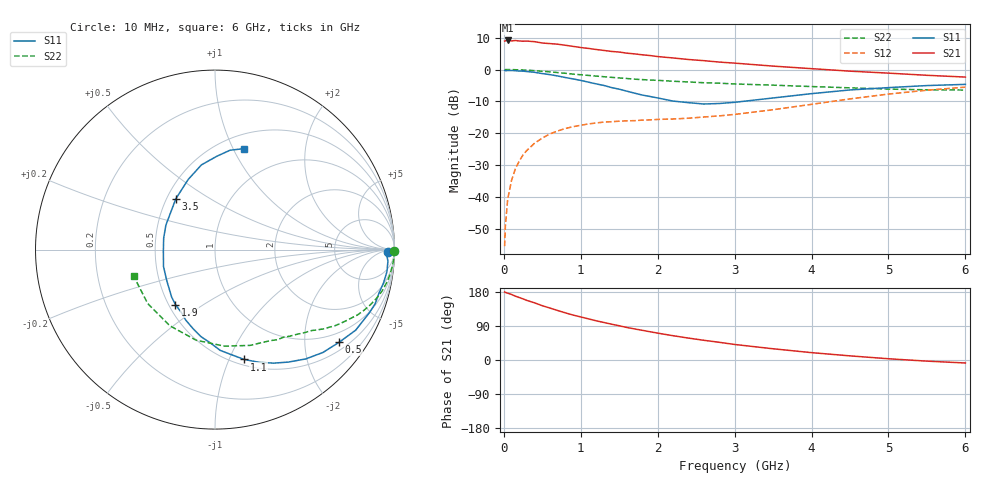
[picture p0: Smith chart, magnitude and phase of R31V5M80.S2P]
! SIEMENS Small Signal Semiconductors
! BFR181
! Si NPN RF Bipolar Junction Transistor in SOT23
! VCE = 1.5 V  IC = 0.8 mA
! Common Emitter S-Parameters:  May  1996
# GHz  S  MA  R  50
!  f  S11  S21  S12  S22
! GHz  MAG  ANG  MAG  ANG  MAG  ANG  MAG  ANG
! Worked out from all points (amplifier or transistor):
!   36 points, 10 MHz to 6 GHz, reference 50 ohm
!   highest |S21| = 9.1 dB at 50 MHz (marker M1)
!   |S21| within 3 dB of that: start of sweep to 1.257 GHz
!   unconditionally stable (mu >= 1): 2.094 GHz to 3.826 GHz
!   at 250 MHz: K = 0.14, MSG = 17.8 dB, |S12| = -26.8 dB
!   at 1.4 GHz: K = 0.72, MSG = 11.0 dB, |S12| = -16.4 dB
!   at 6 GHz: K = 0.91, MSG = 1.6 dB, |S12| = -5.5 dB
!   S11 on the Smith chart (normalised r, x): 10 MHz: 50, -21; 500 MHz: 0.71, -2.86; 1.1 GHz: 0.56, -1.14; 1.9 GHz: 0.54, -0.39; 3.5 GHz: 0.56, +0.36; 6 GHz: 0.64, +1.10
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0.01  0.9665 -0.8  2.79 179.6  0.0017 93.0  0.9993 -0.4
0.02  0.9559 -1.5  2.813 178.4  0.0035 85.1  0.9966 -0.7
0.05  0.9656 -3.8  2.853 176.4  0.0093 88.7  0.9983 -1.8
0.1  0.9659 -7.3  2.81 173.0  0.0182 85.6  0.9962 -3.5
0.15  0.9571 -11.2  2.845 168.4  0.0279 82.0  0.992 -5.4
0.2  0.9458 -14.6  2.803 164.9  0.0366 80.1  0.9872 -7.1
0.3  0.9291 -22.3  2.791 157.2  0.054 75.5  0.976 -10.5
0.4  0.9033 -29.8  2.729 150.8  0.07 70.5  0.9593 -13.9
0.5  0.8632 -36.7  2.602 143.3  0.0842 66.3  0.939 -16.9
0.7  0.7917 -50.3  2.493 130.6  0.1089 58.6  0.8951 -22.3
0.8  0.7481 -56.9  2.399 124.4  0.1189 55.1  0.8728 -24.7
1.1  0.6334 -75.1  2.141 108.6  0.1402 47.1  0.8078 -30.8
1.3  0.5625 -87.0  1.991 99.0  0.1497 43.3  0.7704 -34.1
1.6  0.4572 -105.5  1.803 85.8  0.1568 40.0  0.7229 -38.3
1.9  0.3775 -125.7  1.656 74.6  0.162 39.2  0.6836 -42.4
2.2  0.3198 -147.1  1.516 64.1  0.1675 39.9  0.6542 -46.3
2.6  0.2877 -178.9  1.376 52.0  0.1801 42.9  0.6201 -51.9
3  0.3058 153.5  1.259 41.0  0.1976 46.0  0.5932 -58.8
3.5  0.3579 127.5  1.13 29.6  0.2341 48.6  0.5682 -70.0
4.5  0.4781 99.1  0.942 10.9  0.3459 45.9  0.5157 -101.8
5.5  0.5599 81.4  0.811 -3.0  0.4738 33.4  0.4804 -141.4
6  0.5847 74.1  0.761 -7.9  0.529 25.4  0.4766 -161.9
